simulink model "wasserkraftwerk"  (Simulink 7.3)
settings: Solver=ode23tb  StartTime=0.0  StopTime=1000  MaxStep=0.1  RelTol=1e-4
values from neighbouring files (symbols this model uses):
  A_V0 = 0.518    [dynamic_main.m]    (also in Parameter.m; Parameter_sim.m; static_main.m)
  A_W = pi*5^2    (= 78.5398163397)    [dynamic_main.m]    (also in Parameter.m; Parameter_sim.m; static_main.m)
  c_d = 0.9658    [dynamic_main.m]    (also in Parameter.m = 1; Parameter_sim.m; static_main.m = inv(H3'*H3)*H3'*y3)
  d_F = 2    [dynamic_main.m]    (also in Parameter.m; Parameter_sim.m; static_main.m)
  d_T = 3    [dynamic_main.m]    (also in Parameter.m; Parameter_sim.m; static_main.m)
  d_Turb = 5.35    [dynamic_main.m]    (also in Parameter.m; Parameter_sim.m; static_main.m)
  g = 9.81    [dynamic_main.m]    (also in Parameter.m; Parameter_sim.m; static_main.m)
  h_R = 413    [dynamic_main.m]    (also in Parameter.m; Parameter_sim.m; static_main.m)
  h_W0 = 390    [dynamic_main.m]    (also in Parameter.m; Parameter_sim.m; static_main.m)
  h_W_IC = 413    [dynamic_main.m]    (also in Parameter.m; Parameter_sim.m; static_main.m)
  I_IC = 0    [dynamic_main.m]    (also in Parameter.m; Parameter_sim.m; static_main.m)
  kappa = 8.7000e3    (= 8700)    [dynamic_main.m]    (also in Parameter.m = 1; Parameter_sim.m; static_main.m = inv(H4'*H4)*H4'*y4)
  l_F = 741    [dynamic_main.m]    (also in Parameter.m; Parameter_sim.m; static_main.m)
  L_G = 0.1    [dynamic_main.m]    (also in Parameter.m; Parameter_sim.m; static_main.m)
  L_net = 0.1    [dynamic_main.m]    (also in Parameter_sim.m; static_main.m)
  l_T = 2000    [dynamic_main.m]    (also in Parameter.m; Parameter_sim.m; static_main.m)
  lambda_F = 0.0153    [dynamic_main.m]    (also in Parameter.m = 0.1; Parameter_sim.m; static_main.m = inv(H2'*H2)*H2'*y2)
  lambda_T = 0.0182    [dynamic_main.m]    (also in Parameter.m = 0.1; Parameter_sim.m; static_main.m = inv(H1'*H1)*H1'*y1)
  lambda_W = fminsearch(@(lambda_W)err_wasserschloss(lambda_W,time_bb,V_flw_T_bb,V_flw_F_bb,h_W_bb),lambda_W0)    [dynamic_main.m]    (also in Parameter.m = 10; Parameter_sim.m = 4.0738)
  omega_IC = 0    [dynamic_main.m]    (also in Parameter.m; Parameter_sim.m; static_main.m)
  p_0 = 0    [dynamic_main.m]    (also in Parameter.m; Parameter_sim.m; static_main.m)
  R_G = 10    [dynamic_main.m]    (also in Parameter.m; Parameter_sim.m; static_main.m)
  R_net = 165    [dynamic_main.m]    (also in Parameter_sim.m; static_main.m)
  rho = 1000    [dynamic_main.m]    (also in Parameter.m; Parameter_sim.m; static_main.m)
  sigma_0 = fminsearch(@(sigma_0)err_kompressibilitaet(sigma_0,time_bb,V_flw_F_bb,p_F_bb,x_bb),sigma_0_0)    [dynamic_main.m]    (also in Parameter.m = 1e-15; Parameter_sim.m = 6.279e-10)
  Theta = fminsearch(@(Theta)err_turbine(Theta,time_bb,p_F_bb,x_bb,omega_bb),Theta_0)    [dynamic_main.m]    (also in Parameter.m = 1; Parameter_sim.m = 5499.7)
  v_F_IC = 0    [dynamic_main.m]    (also in Parameter.m; Parameter_sim.m; static_main.m)
  V_F_IC = l_F*pi*d_F^2/4    (= 2327.92015631)    [dynamic_main.m]    (also in Parameter.m; Parameter_sim.m; static_main.m)
  v_T_IC = 0    [dynamic_main.m]    (also in Parameter.m; Parameter_sim.m; static_main.m)
  x_IC = 0    [dynamic_main.m]    (also in Parameter.m; Parameter_sim.m; static_main.m)
undefined symbols (not defined in the file or in its folder): sigbuilder_block

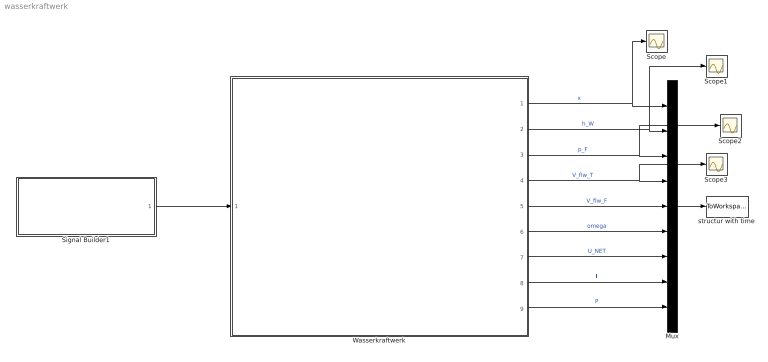
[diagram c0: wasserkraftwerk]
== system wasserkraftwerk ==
  Mux : Mux  Inputs=9
  Scope{,1..3} (4 alike) : Scope
  Signal Builder1 : Subsystem  Tag=STV Subsys  LoadFcn=sigbuilder_block('load');  StartFcn=sigbuilder_block('start');  StopFcn=sigbuilder_block('stop');  ClipboardFcn=sigbuilder_block('clipboard');
  Wasserkraftwerk : Subsystem
  structur with time : ToWorkspace  VariableName=sim_daten  SampleTime=-1  SaveFormat=Structure With Time
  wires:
  Mux/1 -> structur with time/1
  Wasserkraftwerk/1(x) -> Mux/1, Scope/1  "x"
  Wasserkraftwerk/2(h_W) -> Mux/2, Scope1/1  "h_W"
  Wasserkraftwerk/3(p_F) -> Mux/3, Scope2/1  "p_F"
  Wasserkraftwerk/4(V_flw_T) -> Mux/4, Scope3/1  "V_flw_T"
  Wasserkraftwerk/5(V_flw_F) -> Mux/5  "V_flw_F"
  Wasserkraftwerk/6(omega) -> Mux/6  "omega"
  Wasserkraftwerk/7(U_NET) -> Mux/7  "U_NET"
  Wasserkraftwerk/8(I) -> Mux/8  "I"
  Wasserkraftwerk/9(P) -> Mux/9  "P"
  Signal Builder1/1(u) -> Wasserkraftwerk/1(u)

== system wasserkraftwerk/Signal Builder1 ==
  Demux : Demux  Tag=STV Demux  Outputs=1
  FromWs : FromWorkspace  Tag=STV FromWs  VariableName=tuvar  SampleTime=0  SigBuilderData=DataTag0  VnvData=DataTag1
  u : Outport  Tag=STV Outport  OutDataType=sfix(16)  OutScaling=2^0
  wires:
  Demux/1 -> u/1
  FromWs/1 -> Demux/1

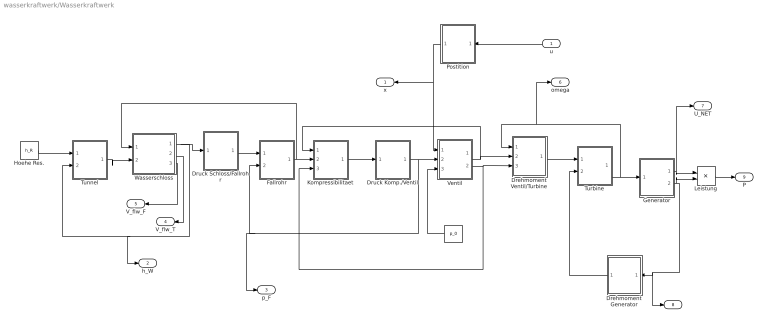
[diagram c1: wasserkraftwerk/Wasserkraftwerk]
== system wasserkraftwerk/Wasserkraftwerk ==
  u : Inport  OutDataType=sfix(16)  OutScaling=2^0
  " " : Constant  Value=p_0  OutDataType=sfix(16)  OutScaling=2^0
  Drehmoment Generator : Subsystem
  Drehmoment Ventil/Turbine : Subsystem
  Druck Komp./Ventil : Subsystem
  Druck Schloss/Fallrohr : Subsystem
  Fallrohr : Subsystem
  Generator : Subsystem
  Hoehe Res. : Constant  Value=h_R  OutDataType=sfix(16)  OutScaling=2^0
  Kompressibilitaet : Subsystem
  Leistung : Product  OutDataType=sfix(16)  OutScaling=2^0
  Postition : Subsystem
  Tunnel : Subsystem
  Turbine : Subsystem
  Ventil : Subsystem
  Wasserschloss : Subsystem
  x : Outport  OutDataType=sfix(16)  OutScaling=2^0
  h_W : Outport  Port=2  OutDataType=sfix(16)  OutScaling=2^0
  p_F : Outport  Port=3  OutDataType=sfix(16)  OutScaling=2^0
  V_flw_T : Outport  Port=4  OutDataType=sfix(16)  OutScaling=2^0
  V_flw_F : Outport  Port=5  OutDataType=sfix(16)  OutScaling=2^0
  omega : Outport  Port=6  OutDataType=sfix(16)  OutScaling=2^0
  U_NET : Outport  Port=7  OutDataType=sfix(16)  OutScaling=2^0
  I : Outport  Port=8  OutDataType=sfix(16)  OutScaling=2^0
  P : Outport  Port=9  OutDataType=sfix(16)  OutScaling=2^0
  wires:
  Hoehe Res./1 -> Tunnel/1(h_R)
  Tunnel/1(v_T) -> Wasserschloss/2(v_T)
  Wasserschloss/1(h_W) -> Druck Schloss/Fallrohr/1(h_W), Tunnel/2(h_W), h_W/1
  Druck Schloss/Fallrohr/1(p_W) -> Fallrohr/1(p_W)
  Fallrohr/1(v_F) -> Kompressibilitaet/2(v_F), Wasserschloss/1(v_F)
  Kompressibilitaet/1(V) -> Druck Komp./Ventil/1(V)
  Druck Komp./Ventil/1(p_F) -> Ventil/2(p_F), Fallrohr/2(p_F), p_F/1
  Ventil/1(A_V) -> Drehmoment Ventil/Turbine/2(A_V), Kompressibilitaet/1(A_V)
  Drehmoment Ventil/Turbine/1(T_T) -> Turbine/1(T_T)
  Turbine/1(w) -> Generator/1(w), Drehmoment Ventil/Turbine/1(w), omega/1
  Generator/2(I) -> Drehmoment Generator/1(I), I/1, Leistung/2
  Ventil/2(v_V) -> Drehmoment Ventil/Turbine/3(v_V), Kompressibilitaet/3(v_V)
  Generator/1(U_NET) -> U_NET/1, Leistung/1
  Leistung/1 -> P/1
  Wasserschloss/2(V_flw_T) -> V_flw_T/1
  Wasserschloss/3(V_flw_T1) -> V_flw_F/1
  " "/1 -> Ventil/3(p_0)
  u/1 -> Postition/1(u)
  Postition/1(x) -> Ventil/1(x), x/1
  Drehmoment Generator/1(T_G) -> Turbine/2(T_G)

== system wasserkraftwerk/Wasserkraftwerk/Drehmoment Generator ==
  I : Inport  OutDataType=sfix(16)  OutScaling=2^0
  Gain : Gain  Gain=kappa  ParameterDataType=sfix(16)  ParameterScaling=2^0  OutDataType=sfix(16)  OutScaling=2^0
  T_G : Outport  OutDataType=sfix(16)  OutScaling=2^0
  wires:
  I/1 -> Gain/1
  Gain/1 -> T_G/1

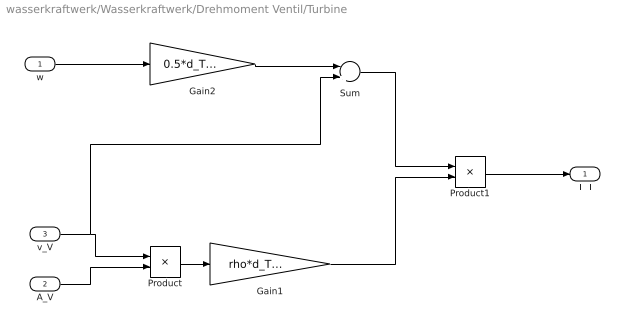
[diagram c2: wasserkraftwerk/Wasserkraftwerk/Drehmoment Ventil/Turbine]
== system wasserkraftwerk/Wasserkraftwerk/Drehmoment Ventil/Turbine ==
  w : Inport  OutDataType=sfix(16)  OutScaling=2^0
  A_V : Inport  Port=2  OutDataType=sfix(16)  OutScaling=2^0
  v_V : Inport  Port=3  OutDataType=sfix(16)  OutScaling=2^0
  Gain1 : Gain  Gain=rho*d_Turb  ParameterDataType=sfix(16)  ParameterScaling=2^0  OutDataType=sfix(16)  OutScaling=2^0
  Gain2 : Gain  Gain=0.5*d_Turb  ParameterDataType=sfix(16)  ParameterScaling=2^0  OutDataType=sfix(16)  OutScaling=2^0
  Product : Product  OutDataType=sfix(16)  OutScaling=2^0
  Product1 : Product  OutDataType=sfix(16)  OutScaling=2^0
  Sum : Sum  Inputs=-+  OutDataType=sfix(16)  OutScaling=2^0
  T_T : Outport  OutDataType=sfix(16)  OutScaling=2^0
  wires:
  Product/1 -> Gain1/1
  w/1 -> Gain2/1
  Gain2/1 -> Sum/1
  v_V/1 -> Product/1, Sum/2
  A_V/1 -> Product/2
  Sum/1 -> Product1/1
  Gain1/1 -> Product1/2
  Product1/1 -> T_T/1

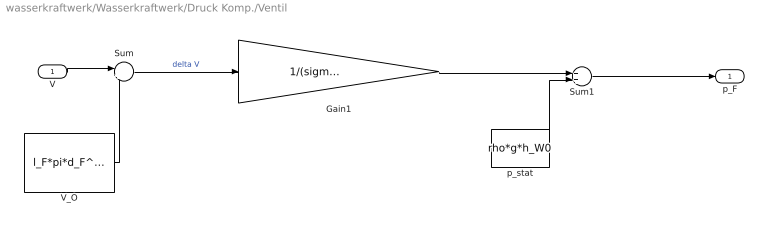
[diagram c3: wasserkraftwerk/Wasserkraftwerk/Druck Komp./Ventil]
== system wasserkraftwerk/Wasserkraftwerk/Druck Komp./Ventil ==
  V : Inport  OutDataType=sfix(16)  OutScaling=2^0
  Gain1 : Gain  Gain=1/(sigma_0 * l_F*pi*d_F^2/4)  ParameterDataType=sfix(16)  ParameterScaling=2^0  OutDataType=sfix(16)  OutScaling=2^0
  Sum : Sum  Inputs=|+-  OutDataType=sfix(16)  OutScaling=2^0
  Sum1 : Sum  OutDataType=sfix(16)  OutScaling=2^0
  V_O : Constant  Value=l_F*pi*d_F^2/4  OutDataType=sfix(16)  OutScaling=2^0
  p_stat : Constant  Value=rho*g*h_W0  OutDataType=sfix(16)  OutScaling=2^0
  p_F : Outport  OutDataType=sfix(16)  OutScaling=2^0
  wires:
  V/1 -> Sum/1
  V_O/1 -> Sum/2
  Sum1/1 -> p_F/1
  p_stat/1 -> Sum1/2
  Sum/1 -> Gain1/1  "delta V"
  Gain1/1 -> Sum1/1

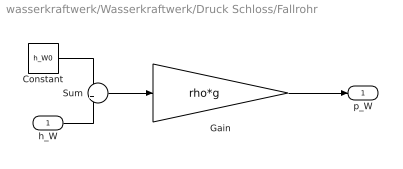
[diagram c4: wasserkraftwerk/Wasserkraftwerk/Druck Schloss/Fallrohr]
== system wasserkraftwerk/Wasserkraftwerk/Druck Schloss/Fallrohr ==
  h_W : Inport  OutDataType=sfix(16)  OutScaling=2^0
  Constant : Constant  Value=h_W0  OutDataType=sfix(16)  OutScaling=2^0
  Gain : Gain  Gain=rho*g  ParameterDataType=sfix(16)  ParameterScaling=2^0  OutDataType=sfix(16)  OutScaling=2^0
  Sum : Sum  Inputs=-+  OutDataType=sfix(16)  OutScaling=2^0
  p_W : Outport  OutDataType=sfix(16)  OutScaling=2^0
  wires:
  Gain/1 -> p_W/1
  Constant/1 -> Sum/1
  h_W/1 -> Sum/2
  Sum/1 -> Gain/1

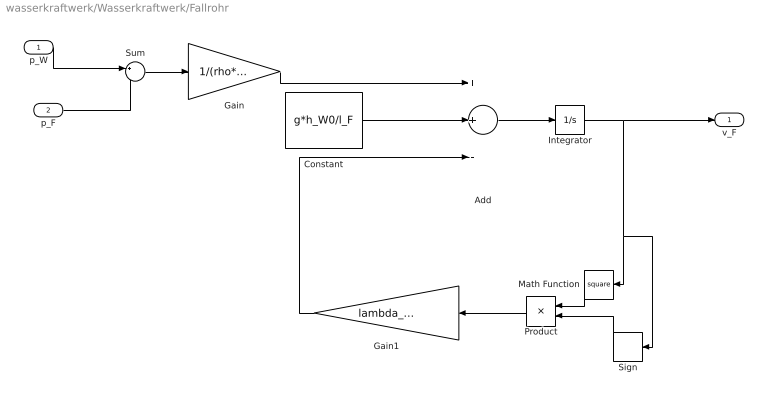
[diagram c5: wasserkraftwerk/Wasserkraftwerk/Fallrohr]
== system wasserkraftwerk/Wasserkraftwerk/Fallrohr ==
  p_W : Inport  OutDataType=sfix(16)  OutScaling=2^0
  p_F : Inport  Port=2  OutDataType=sfix(16)  OutScaling=2^0
  Add : Sum  Inputs=++-  OutDataType=sfix(16)  OutScaling=2^-10
  Constant : Constant  Value=g*h_W0/l_F  OutDataType=sfix(16)  OutScaling=2^0
  Gain : Gain  Gain=1/(rho*l_F)  ParameterDataType=sfix(16)  ParameterScaling=2^0  OutDataType=sfix(16)  OutScaling=2^0
  Gain1 : Gain  Gain=lambda_F/(2*d_F)  ParameterDataType=sfix(16)  ParameterScaling=2^0  OutDataType=sfix(16)  OutScaling=2^0
  Integrator : Integrator  InitialCondition=v_F_IC
  Math Function : Math  Operator=square  OutDataType=sfix(16)  OutScaling=2^0
  Product : Product  OutDataType=sfix(16)  OutScaling=2^0
  Sign : Signum
  Sum : Sum  Inputs=+-  OutDataType=sfix(16)  OutScaling=2^0
  v_F : Outport  OutDataType=sfix(16)  OutScaling=2^0
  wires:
  Product/1 -> Gain1/1
  Sign/1 -> Product/2
  p_W/1 -> Sum/1
  p_F/1 -> Sum/2
  Sum/1 -> Gain/1
  Gain/1 -> Add/1
  Gain1/1 -> Add/3
  Add/1 -> Integrator/1
  Integrator/1 -> v_F/1, Math Function/1, Sign/1
  Math Function/1 -> Product/1
  Constant/1 -> Add/2

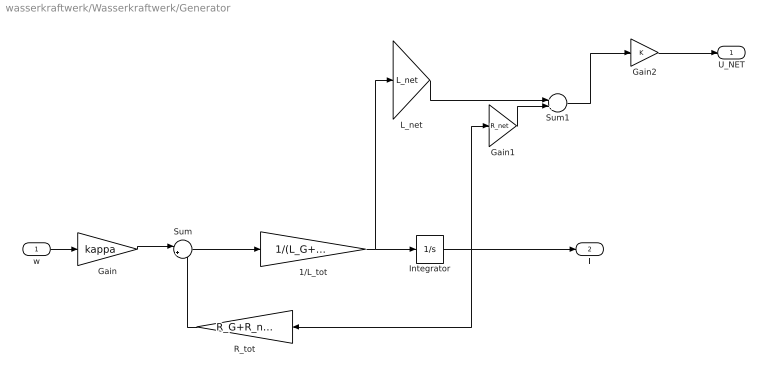
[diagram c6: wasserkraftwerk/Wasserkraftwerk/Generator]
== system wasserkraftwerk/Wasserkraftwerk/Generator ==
  w : Inport  OutDataType=sfix(16)  OutScaling=2^0
  1/L_tot : Gain  Gain=1/(L_G+L_net)  ParameterDataType=sfix(16)  ParameterScaling=2^0  OutDataType=sfix(16)  OutScaling=2^0
  Gain : Gain  Gain=kappa  ParameterDataType=sfix(16)  ParameterScaling=2^0  OutDataType=sfix(16)  OutScaling=2^0
  Gain1 : Gain  Gain=R_net  ParameterDataType=sfix(16)  ParameterScaling=2^0  OutDataType=sfix(16)  OutScaling=2^0
  Gain2 : Gain  ParameterDataType=sfix(16)  ParameterScaling=2^0  OutDataType=sfix(16)  OutScaling=2^0
  Integrator : Integrator  InitialCondition=I_IC
  L_net : Gain  Gain=L_net  ParameterDataType=sfix(16)  ParameterScaling=2^0  OutDataType=sfix(16)  OutScaling=2^0
  R_tot : Gain  Gain=R_G+R_net  ParameterDataType=sfix(16)  ParameterScaling=2^0  OutDataType=sfix(16)  OutScaling=2^0
  Sum : Sum  Inputs=|+-  OutDataType=sfix(16)  OutScaling=2^0
  Sum1 : Sum  OutDataType=sfix(16)  OutScaling=2^0
  U_NET : Outport  OutDataType=sfix(16)  OutScaling=2^0
  I : Outport  Port=2  OutDataType=sfix(16)  OutScaling=2^0
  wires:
  Integrator/1 -> I/1, R_tot/1, Gain1/1
  w/1 -> Gain/1
  Gain/1 -> Sum/1
  Sum/1 -> 1/L_tot/1
  1/L_tot/1 -> Integrator/1, L_net/1
  Gain2/1 -> U_NET/1
  Gain1/1 -> Sum1/2
  R_tot/1 -> Sum/2
  Sum1/1 -> Gain2/1
  L_net/1 -> Sum1/1

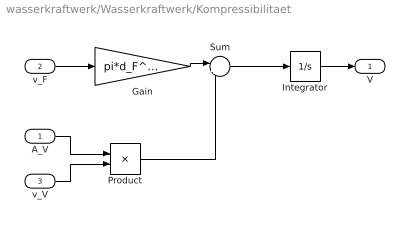
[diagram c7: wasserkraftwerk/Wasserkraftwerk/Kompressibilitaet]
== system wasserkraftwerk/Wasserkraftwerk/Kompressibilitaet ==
  A_V : Inport  OutDataType=sfix(16)  OutScaling=2^0
  v_F : Inport  Port=2  OutDataType=sfix(16)  OutScaling=2^0
  v_V : Inport  Port=3  OutDataType=sfix(16)  OutScaling=2^0
  Gain : Gain  Gain=pi*d_F^2/4  ParameterDataType=sfix(16)  ParameterScaling=2^0  OutDataType=sfix(16)  OutScaling=2^0
  Integrator : Integrator  InitialCondition=V_F_IC
  Product : Product  OutDataType=sfix(16)  OutScaling=2^0
  Sum : Sum  Inputs=|+-  OutDataType=sfix(16)  OutScaling=2^0
  V : Outport  OutDataType=sfix(16)  OutScaling=2^0
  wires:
  v_F/1 -> Gain/1
  Gain/1 -> Sum/1
  A_V/1 -> Product/1
  v_V/1 -> Product/2
  Product/1 -> Sum/2
  Sum/1 -> Integrator/1
  Integrator/1 -> V/1

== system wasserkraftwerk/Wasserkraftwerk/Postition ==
  u : Inport  OutDataType=sfix(16)  OutScaling=2^0
  Integrator : Integrator  InitialCondition=x_IC  LimitOutput=on  UpperSaturationLimit=1  LowerSaturationLimit=0
  x : Outport  OutDataType=sfix(16)  OutScaling=2^0
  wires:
  u/1 -> Integrator/1
  Integrator/1 -> x/1

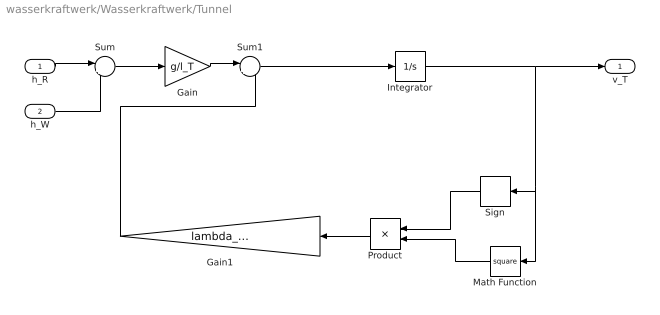
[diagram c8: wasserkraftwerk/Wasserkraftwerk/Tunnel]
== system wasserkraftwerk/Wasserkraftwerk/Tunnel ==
  h_R : Inport  OutDataType=sfix(16)  OutScaling=2^0
  h_W : Inport  Port=2  OutDataType=sfix(16)  OutScaling=2^0
  Gain : Gain  Gain=g/l_T  ParameterDataType=sfix(16)  ParameterScaling=2^0  OutDataType=sfix(16)  OutScaling=2^0
  Gain1 : Gain  Gain=lambda_T/(2*d_T)  ParameterDataType=sfix(16)  ParameterScaling=2^0  OutDataType=sfix(16)  OutScaling=2^0
  Integrator : Integrator  InitialCondition=v_T_IC
  Math Function : Math  Operator=square  OutDataType=sfix(16)  OutScaling=2^0
  Product : Product  OutDataType=sfix(16)  OutScaling=2^0
  Sign : Signum
  Sum : Sum  Inputs=|+-  OutDataType=sfix(16)  OutScaling=2^0
  Sum1 : Sum  Inputs=|+-  OutDataType=sfix(16)  OutScaling=2^0
  v_T : Outport  OutDataType=sfix(16)  OutScaling=2^0
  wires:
  h_R/1 -> Sum/1
  h_W/1 -> Sum/2
  Sum/1 -> Gain/1
  Gain/1 -> Sum1/1
  Sum1/1 -> Integrator/1
  Integrator/1 -> v_T/1, Sign/1, Math Function/1
  Product/1 -> Gain1/1
  Sign/1 -> Product/1
  Math Function/1 -> Product/2
  Gain1/1 -> Sum1/2

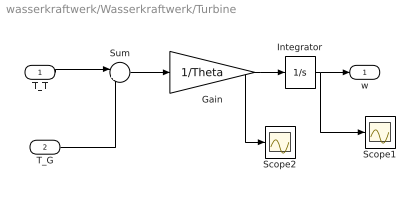
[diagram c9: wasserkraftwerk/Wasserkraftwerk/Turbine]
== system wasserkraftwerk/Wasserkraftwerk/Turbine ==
  T_T : Inport  OutDataType=sfix(16)  OutScaling=2^0
  T_G : Inport  Port=2  OutDataType=sfix(16)  OutScaling=2^0
  Gain : Gain  Gain=1/Theta  ParameterDataType=sfix(16)  ParameterScaling=2^0  OutDataType=sfix(16)  OutScaling=2^0
  Integrator : Integrator  InitialCondition=omega_IC
  Scope1 : Scope
  Scope2 : Scope
  Sum : Sum  Inputs=|+-  OutDataType=sfix(16)  OutScaling=2^0
  w : Outport  OutDataType=sfix(16)  OutScaling=2^0
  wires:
  T_T/1 -> Sum/1
  T_G/1 -> Sum/2
  Sum/1 -> Gain/1
  Gain/1 -> Integrator/1, Scope2/1
  Integrator/1 -> w/1, Scope1/1

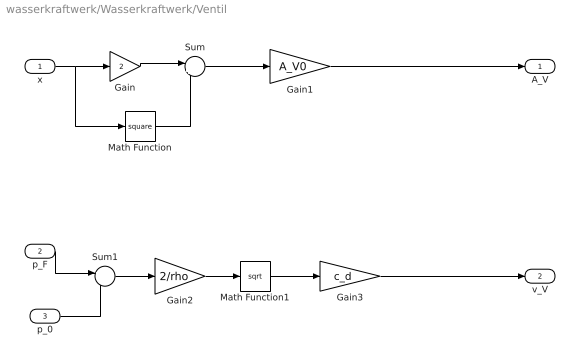
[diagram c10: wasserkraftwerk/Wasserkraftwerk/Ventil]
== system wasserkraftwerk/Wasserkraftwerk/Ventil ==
  x : Inport  OutDataType=sfix(16)  OutScaling=2^0
  p_F : Inport  Port=2  OutDataType=sfix(16)  OutScaling=2^0
  p_0 : Inport  Port=3  OutDataType=sfix(16)  OutScaling=2^0
  Gain : Gain  Gain=2  ParameterDataType=sfix(16)  ParameterScaling=2^0  OutDataType=sfix(16)  OutScaling=2^0
  Gain1 : Gain  Gain=A_V0  ParameterDataType=sfix(16)  ParameterScaling=2^0  OutDataType=sfix(16)  OutScaling=2^0
  Gain2 : Gain  Gain=2/rho  ParameterDataType=sfix(16)  ParameterScaling=2^0  OutDataType=sfix(16)  OutScaling=2^0
  Gain3 : Gain  Gain=c_d  ParameterDataType=sfix(16)  ParameterScaling=2^0  OutDataType=sfix(16)  OutScaling=2^0
  Math Function : Math  Operator=square  OutDataType=sfix(16)  OutScaling=2^0
  Math Function1 : Math  Operator=sqrt  OutDataType=sfix(16)  OutScaling=2^0
  Sum : Sum  Inputs=|+-  OutDataType=sfix(16)  OutScaling=2^0
  Sum1 : Sum  Inputs=+-  OutDataType=sfix(16)  OutScaling=2^0
  A_V : Outport  OutDataType=sfix(16)  OutScaling=2^0
  v_V : Outport  Port=2  OutDataType=sfix(16)  OutScaling=2^0
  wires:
  x/1 -> Gain/1, Math Function/1
  Gain/1 -> Sum/1
  Math Function/1 -> Sum/2
  Sum/1 -> Gain1/1
  Gain1/1 -> A_V/1
  p_F/1 -> Sum1/1
  p_0/1 -> Sum1/2
  Sum1/1 -> Gain2/1
  Gain2/1 -> Math Function1/1
  Math Function1/1 -> Gain3/1
  Gain3/1 -> v_V/1

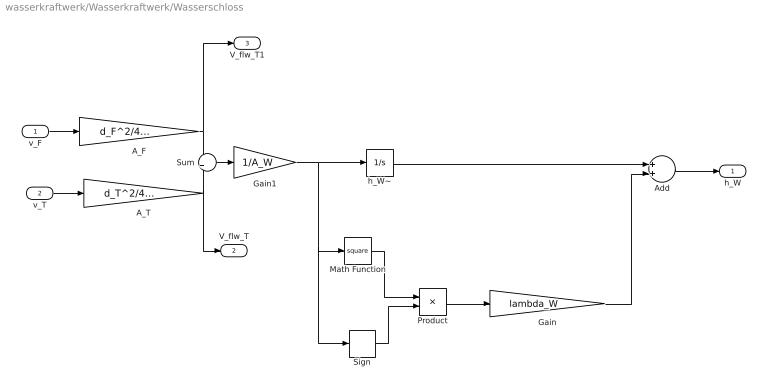
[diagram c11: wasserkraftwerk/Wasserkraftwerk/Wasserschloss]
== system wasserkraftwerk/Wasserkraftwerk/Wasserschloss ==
  v_F : Inport  OutDataType=sfix(16)  OutScaling=2^0
  v_T : Inport  Port=2  OutDataType=sfix(16)  OutScaling=2^0
  A_F : Gain  Gain=d_F^2/4*pi  ParameterDataType=sfix(16)  ParameterScaling=2^0  OutDataType=sfix(16)  OutScaling=2^0
  A_T : Gain  Gain=d_T^2/4*pi  ParameterDataType=sfix(16)  ParameterScaling=2^0  OutDataType=sfix(16)  OutScaling=2^0
  Add : Sum  OutDataType=sfix(16)  OutScaling=2^-10
  Gain : Gain  Gain=lambda_W  ParameterDataType=sfix(16)  ParameterScaling=2^0  OutDataType=sfix(16)  OutScaling=2^0
  Gain1 : Gain  Gain=1/A_W  ParameterDataType=sfix(16)  ParameterScaling=2^0  OutDataType=sfix(16)  OutScaling=2^0
  Math Function : Math  Operator=square  OutDataType=sfix(16)  OutScaling=2^0
  Product : Product  OutDataType=sfix(16)  OutScaling=2^0
  Sign : Signum
  Sum : Sum  Inputs=-+  OutDataType=sfix(16)  OutScaling=2^0
  h_W~ : Integrator  InitialCondition=h_W_IC
  h_W : Outport  OutDataType=sfix(16)  OutScaling=2^0
  V_flw_T : Outport  Port=2  OutDataType=sfix(16)  OutScaling=2^0
  V_flw_T1 : Outport  Port=3  OutDataType=sfix(16)  OutScaling=2^0
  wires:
  Product/1 -> Gain/1
  v_T/1 -> A_T/1
  v_F/1 -> A_F/1
  A_F/1 -> Sum/1, V_flw_T1/1
  A_T/1 -> Sum/2, V_flw_T/1
  Sum/1 -> Gain1/1
  Gain1/1 -> h_W~/1, Math Function/1, Sign/1
  Math Function/1 -> Product/1
  Sign/1 -> Product/2
  h_W~/1 -> Add/1
  Add/1 -> h_W/1
  Gain/1 -> Add/2
